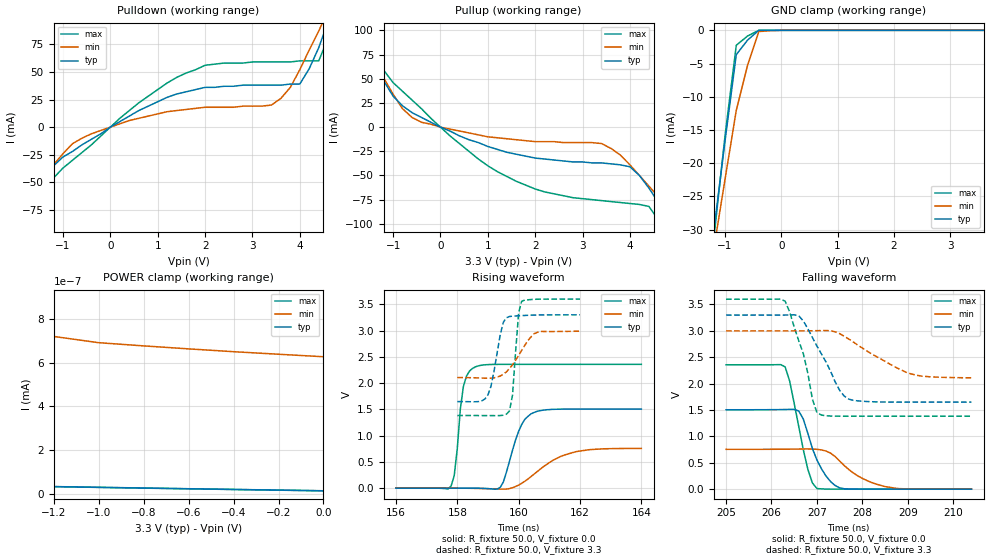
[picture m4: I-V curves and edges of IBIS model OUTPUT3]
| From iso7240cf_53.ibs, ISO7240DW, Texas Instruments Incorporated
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[Model]   OUTPUT3
Model_type   3-state
| Signals   OUT
Vmeas = 2.2V   |Reference voltage for timing measurements
Cref = 15pF   |Timing specification test load capacitance value
Vref = 0   |Timing specification test load voltage; GND
| variable   typ   min   max
C_comp   2.1pF   1.7pF   2.5pF
|   typ   min   max
[Temperature Range]   25.0   -40   125
[Voltage range]   3.3V   3.0V   3.6V
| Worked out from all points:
|   slope of the pulldown table from 0 to 0.495 V, typ, clamps not added: 40 ohm
|   slope of the pullup table from 0 to 0.495 V, typ, clamps not added: 45.4 ohm
|   GND clamp passes 1 mA (typ) near -0.54 V on its own axis
|   POWER clamp passes 1 mA (typ) near -2.27 V on its own axis
|   rising waveform, R_fixture 50.0, V_fixture 0.0: 20-80 % time 494ps typ, 1.13ns min, 242ps max; typ from 0 V to 1.5 V
|   falling waveform, R_fixture 50.0, V_fixture 0.0: 20-80 % time 416ps typ, 716ps min, 336ps max; typ from 1.5 V to 0 V
|   rising waveform, R_fixture 50.0, V_fixture 3.3: 20-80 % time 308ps typ, 597ps min, 168ps max; typ from 1.65 V to 3.3 V
|   falling waveform, R_fixture 50.0, V_fixture 3.3: 20-80 % time 592ps typ, 1.04ns min, 405ps max; typ from 3.3 V to 1.65 V
[Pulldown]
|   Voltage  I(typ)   I(min)   I(max)
-3.6V     -213mA     -167mA     -286mA
-2.2V     -106mA     -89mA      -137mA
-1.8V     -76mA      -66mA      -95mA
-1.2V     -35mA      -34mA      -46mA
-600mV    -16mA      -10mA      -23mA
2V        36mA       18mA       56mA
3.4V      38mA       20mA       59mA
4V        39mA       52mA       60mA
4.4V      72mA       87mA       60mA
4.6V      96mA       106mA      81mA
4.8V      120mA      124mA      106mA
7.5V      465mA      379mA      575mA
[Pullup]
|   Voltage   I(typ)  I(min)  I(max)
| Note that the[Pullup]voltage table is referenced to Vcc
| and is calculated using Vtable=Vcc - Vmeasured.
-3.6V     345mA      272mA      457mA
-2V       144mA      123mA      182mA
-1.5V     83mA       78mA       100mA
-1.2V     48mA       51mA       59mA
-600mV    15mA       10mA       28mA
800mV     -16mA      -8mA       -33mA
2V        -32mA      -15mA      -64mA
3.4V      -37mA      -17mA      -76mA
4V        -41mA      -39mA      -79mA
4.4V      -63mA      -61mA      -82mA
5V        -108mA     -95mA      -134mA
7.2V      -281mA     -221mA     -373mA
[GND_clamp]
|   Voltage   I(typ)   I(min)   I(max)
| Outputs in High Impedance (off)
-3.6V     -213mA     -167.2mA   -285.4mA
-1.2V     -30.16mA   -32.94mA   -31.43mA
-1.1V     -23.41mA   -27.68mA   -23.65mA
-1V       -16.66mA   -22.42mA   -15.87mA
-800mV    -3.66mA    -12.05mA   -2.249mA
-600mV    -1.479mA   -5.279mA   -861.1uA
-400mV    -1.657uA   -187.7uA   -4.797uA
0V        -40.79pA   -10.95nA   -39.6pA
3.6V      17.57pA    663pA      12.68pA
[POWER_clamp]
|   Voltage  I(typ)   I(min)   I(max)
| Note that the [POWER_clamp] voltage table is referenced to Vcc
| and is calculated using Vtable = Vcc - Vmeasured.
| Outputs in Tri-state.
-3.6V     130.9mA    132.2mA    129.3mA
-2.2V     594.7uA    10.13mA    942.3pA
-2.1V     8.158nA    6.126mA    495.1pA
-2V       5.434nA    2.119mA    47.98pA
-1.8V     1.376nA    388.9uA    43.35pA
-1.7V     41.24pA    194.6uA    41.32pA
-1.5V     37.53pA    132.3nA    37.35pA
-1.4V     35.76pA    755.1pA    35.42pA
-1.2V     32.25pA    720.1pA    31.79pA
-1V       28.85pA    691.4pA    28.37pA
-400mV    19.15pA    650.1pA    18.72pA
0V        12.94pA    627pA      12.68pA
[Ramp]
|   typ   min   max
dV/dt_r   0.903V/0.494ns   0.454V/1.13ns   1.414V/0.242ns
dV/dt_f   0.903V/0.416ns   0.453V/0.717ns  1.414V/0.336ns
R_load = 50
[Rising Waveform]
R_fixture = 50.0
V_fixture = 0.0
C_fixture = 0p
L_fixture = 0n
|   V(typ)   V(min)   V(max)
156ns     489.7pV    12.09nV    431.9pV
157.8ns   17.01uV    282.3uV    42.76mV
157.9ns   27.86uV    217.4uV    238.3mV
158.2ns   89.93uV    -788.4uV   1.94V
158.6ns   -99.63uV   -4.419mV   2.312V
159.4ns   15.91mV    -17.3mV    2.357V
160ns     1.083V     58.82mV    2.357V
160.5ns   1.441V     266mV      2.357V
161.9ns   1.506V     698.7mV    2.357V
164ns     1.505V     756mV      2.357V
[Falling Waveform]
R_fixture = 50.0
V_fixture = 0.0
C_fixture = 0p
L_fixture = 0n
|   V(typ)   V(min)   V(max)
205ns     1.505V     755.2mV    2.357V
206.3ns   1.51V      757.4mV    2.318V
206.4ns   1.512V     758.3mV    2.047V
206.6ns   1.481V     760.6mV    1.187V
206.8ns   1.057V     762mV      375.6mV
207ns     553.1mV    755.1mV    12.03mV
207.3ns   143.1mV    683mV      796.9uV
207.6ns   7.515mV    447.7mV    36.71uV
208.5ns   197.3uV    48.97mV    -2.819uV
210.4ns   -4.04uV    324.3uV    303.2nV
[Rising Waveform]
R_fixture = 50.0
V_fixture = 3.3
V_fixture_min = 3.0
V_fixture_max = 3.6
C_fixture = 0p
L_fixture = 0n
|   V(typ)   V(min)  V(max)
158ns     1.649V     2.106V     1.383V
159ns     1.774V     2.093V     1.382V
159.1ns   1.943V     2.094V     1.382V
159.5ns   3.156V     2.171V     1.389V
159.7ns   3.268V     2.277V     1.468V
159.8ns   3.274V     2.348V     1.768V
160ns     3.282V     2.527V     3.341V
160.1ns   3.285V     2.625V     3.559V
160.6ns   3.296V     2.964V     3.597V
162ns     3.3V       2.989V     3.6V
[Falling Waveform]
R_fixture = 50.0
V_fixture = 3.3
V_fixture_min = 3.0
V_fixture_max = 3.6
C_fixture = 0p
L_fixture = 0n
|   V(typ)   V(min)  V(max)
205ns     3.3V       3V         3.6V
206.3ns   3.3V       3V         3.563V
206.6ns   3.286V     3V         2.812V
206.7ns   3.187V     3V         2.569V
206.9ns   2.874V     3.002V     1.705V
207.1ns   2.561V     3.006V     1.404V
207.5ns   1.872V     2.947V     1.383V
207.7ns   1.707V     2.846V     1.383V
209ns     1.65V      2.201V     1.383V
210.4ns   1.65V      2.11V      1.383V
